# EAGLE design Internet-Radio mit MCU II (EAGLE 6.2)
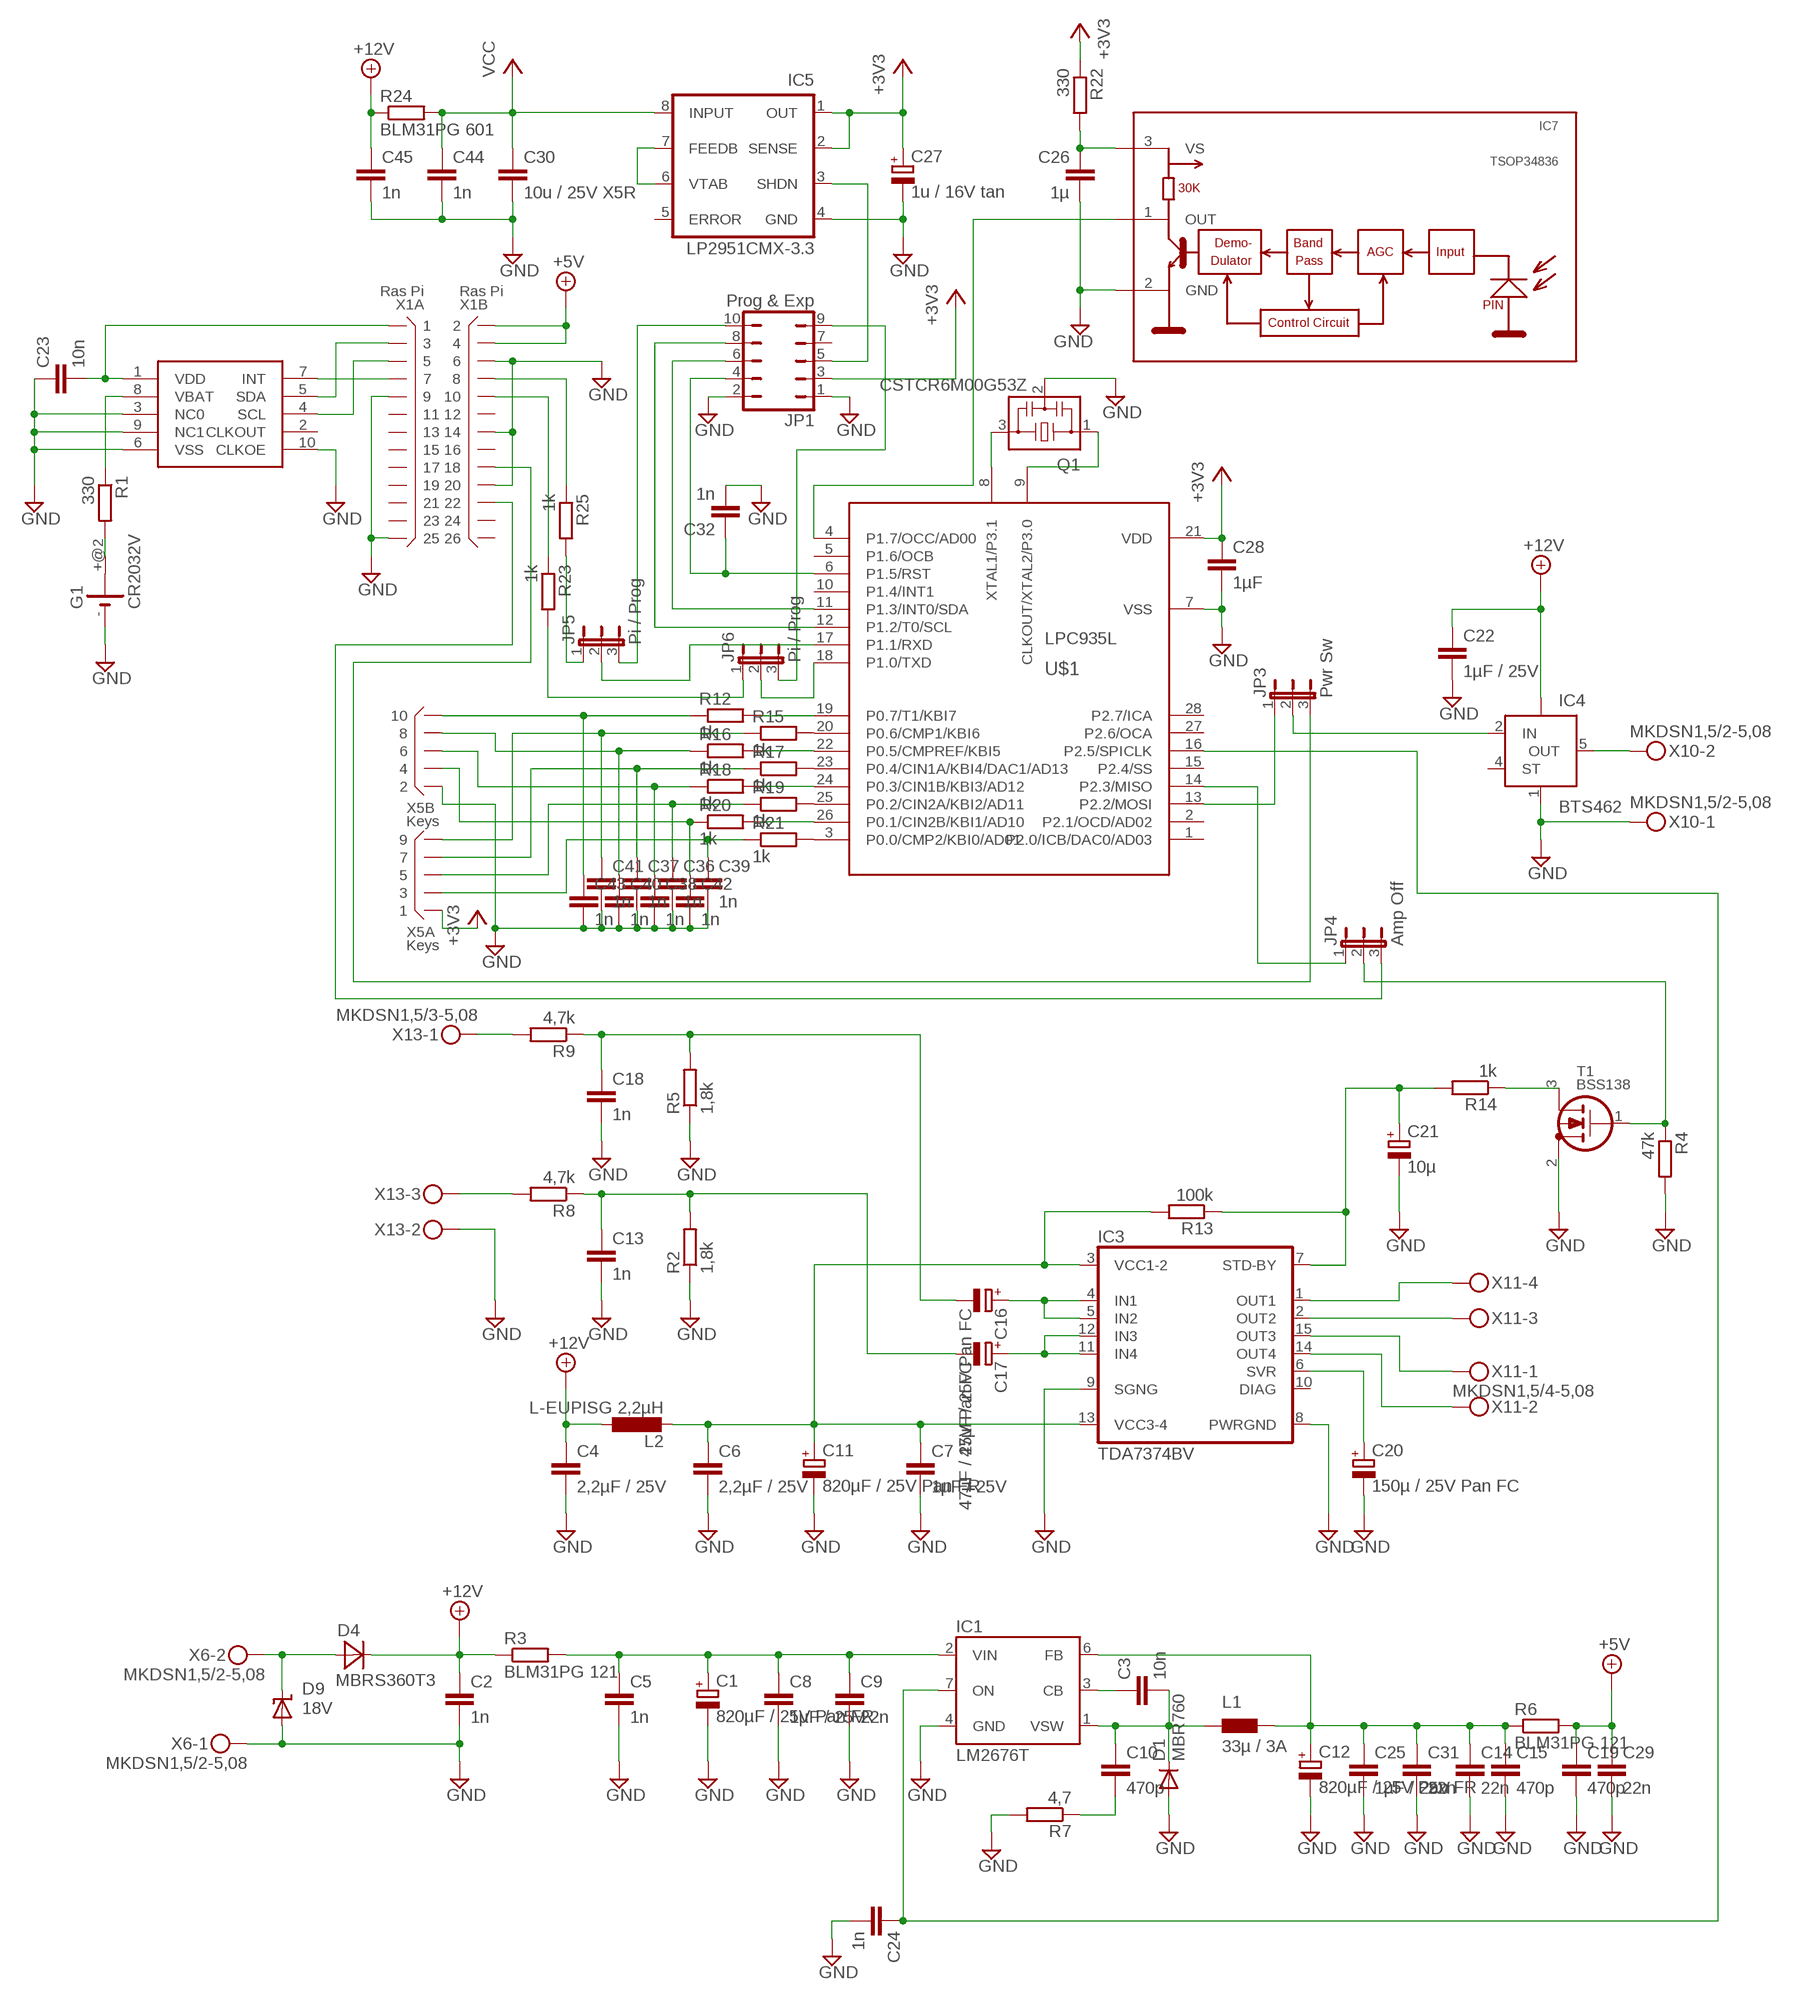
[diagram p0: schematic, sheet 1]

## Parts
C1  820µF / 25V Pan FR  CPOL-EUTT5D10  [TT5D10]
C2  1n  C-EUC0805  [C0805]
C3  10n  C-EUC0805  [C0805]
C4  2,2µF / 25V  C-EUC0805  [C0805]
C5  1n  C-EUC0805  [C0805]
C6  2,2µF / 25V  C-EUC0805  [C0805]
C7  1µF / 25V  C-EUC0805  [C0805]
C8  1µF / 25V  C-EUC0805  [C0805]
C9  22n  C-EUC0805  [C0805]
C10  470p  C-EUC0805  [C0805]
C11  820µF / 25V Pan FR  CPOL-EUTT5D10  [TT5D10]
C12  820µF / 25V Pan FR  CPOL-EUTT5D10  [TT5D10]
C13  1n  C-EUC0805  [C0805]
C14  22n  C-EUC0805  [C0805]
C15  470p  C-EUC0805  [C0805]
C16  47µF / 25V Pan FC  CPOL-EUE2.5-5  [E2,5-5]
C17  47µF / 25V Pan FC  CPOL-EUE2.5-5  [E2,5-5]
C18  1n  C-EUC0805  [C0805]
C19  470p  C-EUC0805  [C0805]
C20  150µ / 25V Pan FC  CPOL-EUE3.5-8  [E3,5-8]
C21  10µ  CPOL-EUE2.5-5  [E2,5-5]
C22  1µF / 25V  C-EUC0805  [C0805]
C23  10n  C-EUC0805  [C0805]
C24  1n  C-EUC0805  [C0805]
C25  1µF / 25V  C-EUC0805  [C0805]
C26  1µ  C-EUC0805  [C0805]
C27  1u / 16V tan  CPOL-EUCT3216  [CT3216]
C28  1µF  C-EUC0805  [C0805]
C29  22n  C-EUC0805  [C0805]
C30  10u / 25V X5R  C-EUC1206  [C1206]
C31  22n  C-EUC0805  [C0805]
C32  1n  C-EUC0805  [C0805]
C36  1n  C-EUC0603  [C0603]
C37  1n  C-EUC0603  [C0603]
C38  1n  C-EUC0603  [C0603]
C39  1n  C-EUC0603  [C0603]
C40  1n  C-EUC0603  [C0603]
C41  1n  C-EUC0603  [C0603]
C42  1n  C-EUC0603  [C0603]
C43  1n  C-EUC0603  [C0603]
C44  1n  C-EUC0805  [C0805]
C45  1n  C-EUC0805  [C0805]
D1  MBR760  DIODE-TO220V  [TO220ACS]
D4  MBRS360T3  [SMC]
D9  18V  SUPPRESSOR-SMBJ  [SMBJ]
G1  CR2032V  [CR2032V]
IC1  LM2676T  [TO220-7]
IC3  TDA7374BV  [MULTIWATT-15V]
IC4  BTS462  BTS428L2  [TO252-5-11]
IC5  LP2951CMX-3.3  [SO-08]
IC7  TSOP34836  [TSOP348]
JP1  Prog & Exp  JP5Q  [JP5Q]
JP3  Pwr Sw  JP2E  [JP2]
JP4  Amp Off  JP2E  [JP2]
JP5  Pi / Prog  JP2E  [JP2]
JP6  Pi / Prog  JP2E  [JP2]
L1  33µ / 3A  PIS4728  [PIS4728]
L2  L-EUPISG 2,2µH  L-EUPISG  [PISG]
Q1  CSTCR6M00G53Z  [CSTCR6M]
R1  330  R-EU_R1206  [R1206]
R2  1,8k  R-EU_R1206  [R1206]
R3  BLM31PG 121  R-EU_R1206  [R1206]
R4  47k  R-EU_R1206  [R1206]
R5  1,8k  R-EU_R1206  [R1206]
R6  BLM31PG 121  R-EU_R1206  [R1206]
R7  4,7  R-EU_R1206  [R1206]
R8  4,7k  R-EU_R1206  [R1206]
R9  4,7k  R-EU_R1206  [R1206]
R12  1k  R-EU_R1206  [R1206]
R13  100k  R-EU_R1206  [R1206]
R14  1k  R-EU_R1206  [R1206]
R15  1k  R-EU_R1206  [R1206]
R16  1k  R-EU_R1206  [R1206]
R17  1k  R-EU_R1206  [R1206]
R18  1k  R-EU_R1206  [R1206]
R19  1k  R-EU_R1206  [R1206]
R20  1k  R-EU_R1206  [R1206]
R21  1k  R-EU_R1206  [R1206]
R22  330  R-EU_R1206  [R1206]
R23  1k  R-EU_R1206  [R1206]
R24  BLM31PG 601  R-EU_R1206  [R1206]
R25  1k  R-EU_R1206  [R1206]
T1  BSS138  [SOT23]
U$1  LPC935L  [PLCC28]
U$4  RV3029-C2  [MC_RTC]
X1  Ras Pi  X13X2  [X26N-IDC]
X5  Keys  X05X2  [X10N-IDC]
X6  MKDSN1,5/2-5,08  [MKDSN1,5/2-5,08]
X10  MKDSN1,5/2-5,08  [MKDSN1,5/2-5,08]
X11  MKDSN1,5/4-5,08  [MKDSN1,5/4-5,08]
X13  MKDSN1,5/3-5,08  [MKDSN1,5/3-5,08]

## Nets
+3V3: C27.+ C28.1 IC5.1(OUT) IC5.2(SENSE) JP1.3 R22.1 U$1.21(VDD) X5.1
+5V: C19.1 C29.1 R6.2 X1.2 X1.4
+12V: C2.1 C4.1 C22.1 C45.1 D4.C IC4.TAB(VBB) L2.1 R3.1 R24.1
GND: C1.- C2.2 C4.2 C5.2 C6.2 C7.2 C8.2 C9.2 C11.- C12.- C13.2 C14.2 C15.2 C18.2 C19.2 C20.- C21.- C22.2 C23.1 C24.2 C25.2 C26.2 C27.- C28.2 C29.2 C30.2 C31.2 C32.2 C36.2 C37.2 C38.2 C39.2 C40.2 C41.2 C42.2 C43.2 C44.2 C45.2 D1.A D9.A G1.- IC1.4(GND) IC3.8(PWRGND) IC3.9(SGNG) IC4.1(GND) IC5.4(GND) IC7.2(GND) JP1.1 JP1.2 Q1.2 R2.1 R4.2 R5.1 R7.2 T1.2(S) U$1.7(VSS) U$4.3(NC0) U$4.6(VSS) U$4.9(NC1) U$4.10(CLKOE) X1.6 X1.9 X1.14 X1.20 X1.25 X5.2 X6.1 X10.1 X13.2
N$1: C1.+ C5.1 C8.1 C9.1 IC1.2(VIN) R3.2
N$2: C3.2 C10.1 D1.C IC1.1(VSW) L1.P$1
N$3: IC3.1(OUT1) X11.4
N$4: C3.1 IC1.3(CB)
N$5: IC3.2(OUT2) X11.3
N$6: IC3.15(OUT3) X11.1
N$7: IC3.14(OUT4) X11.2
N$8: C6.1 C7.1 C11.+ IC3.3(VCC1-2) IC3.13(VCC3-4) L2.2 R13.2
N$9: D4.A D9.C X6.2
N$10: C20.+ IC3.6(SVR)
N$11: G1.+@2(+) R1.2
N$12: C16.- C18.1 R5.2 R9.1
N$13: R9.2 X13.1
N$14: C13.1 C17.- R2.2 R8.1
N$15: C10.2 R7.1
N$16: R8.2 X13.3
N$17: C12.+ C14.1 C15.1 C25.1 C31.1 IC1.6(FB) L1.P$2 R6.1
N$18: C21.+ IC3.7(STD-BY) R13.1 R14.2
N$20: IC4.5(OUT) X10.2
N$23: R14.1 T1.3(D)
N$24: C16.+ IC3.4(IN1) IC3.5(IN2)
N$25: JP4.2 R4.1 T1.1(G)
N$26: C17.+ IC3.11(IN4) IC3.12(IN3)
N$27: JP3.1 U$1.13(P2.2/MOSI)
N$28: C24.1 IC1.7(ON) U$1.16(P2.5/SPICLK)
N$29: R1.1 U$4.8(VBAT)
N$30: Q1.3 U$1.8(XTAL1/P3.1)
N$31: Q1.1 U$1.9(CLKOUT/XTAL2/P3.0)
N$32: R12.2 U$1.19(P0.7/T1/KBI7)
N$33: R15.2 U$1.20(P0.6/CMP1/KBI6)
N$34: R16.2 U$1.22(P0.5/CMPREF/KBI5)
N$35: R18.2 U$1.24(P0.3/CIN1B/KBI3/AD12)
N$36: R20.2 U$1.26(P0.1/CIN2B/KBI1/AD10)
N$37: R21.2 U$1.3(P0.0/CMP2/KBI0/AD01)
N$38: R19.2 U$1.25(P0.2/CIN2A/KBI2/AD11)
N$39: R17.2 U$1.23(P0.4/CIN1A/KBI4/DAC1/AD13)
N$40: C26.1 IC7.3(VS) R22.2
N$41: IC5.6(VTAB) IC5.7(FEEDB)
N$42: C38.1 R18.1 X5.6
N$43: C36.1 R19.1 X5.5
N$44: C42.1 R20.1 X5.4
N$45: C39.1 R21.1 X5.3
N$46: C43.1 R12.1 X5.10
N$47: C41.1 R15.1 X5.9
N$48: C40.1 R16.1 X5.8
N$49: C37.1 R17.1 X5.7
N$50: C23.2 U$4.1(VDD) X1.1
N$51: JP5.1 R25.2
N$52: IC7.1(OUT) U$1.4(P1.7/OCC/AD00)
N$53: JP6.1 R23.2
N$54: R23.1 X1.10
N$55: R25.1 X1.8
N$56: C32.1 JP1.4 U$1.6(P1.5/RST)
N$57: IC5.3(SHDN) JP1.5
N$58: IC4.2(IN) JP3.2
N$59: JP3.3 X1.18
N$60: JP4.3 X1.22
N$61: JP6.2 U$1.18(P1.0/TXD)
N$62: JP4.1 U$1.14(P2.3/MISO)
N$63: JP5.2 U$1.17(P1.1/RXD)
P1.0: JP1.9 JP6.3
P1.1: JP1.10 JP5.3
P1.2: JP1.8 U$1.12(P1.2/T0/SCL)
P1.3: JP1.6 U$1.11(P1.3/INT0/SDA)
P1.4: U$4.5(SDA) X1.3
P1.5: U$4.4(SCL) X1.5
P1.6: U$4.7(INT) X1.7
VCC: C30.1 C44.1 IC5.8(INPUT) R24.2
Unconnected: G1.+ IC3.10(DIAG) IC4.4(ST) IC5.5(ERROR) JP1.7 U$1.1(P2.0/ICB/DAC0/AD03) U$1.2(P2.1/OCD/AD02) U$1.5(P1.6/OCB) U$1.10(P1.4/INT1) U$1.15(P2.4/SS) U$1.27(P2.6/OCA) U$1.28(P2.7/ICA) U$4.2(CLKOUT) X1.11 X1.12 X1.13 X1.15 X1.16 X1.17 X1.19 X1.21 X1.23 X1.24 X1.26

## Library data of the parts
C1 C11 C12 C16 C17 C20 C21 C27 = rcl:CPOL-EU: POLARIZED CAPACITOR, European symbol
C2-C10 C13-C15 C18 C19 C22-C26 C28-C32 C36-C45 = rcl:C-EU: CAPACITOR, European symbol
D1 = diode:DIODE-: DIODE
D4 = diode:MBRS360T3: Surface Mount Schottky Power Rectifier
D9 = diode:SUPPRESSOR-: Suppressor diode
G1 = battery:CR2032V: LI BATTERY Varta
IC1 = v-reg-3:LM2676: National Semiconductor 3.0A "Simple Switcher"(c) 260kHz, Vout 1.2-37V, Vin 40V, 150mOhm DMOS switch, 50µA standby current
IC3 = st-tda737X:TDA7374B
IC4 = infineon:BTS428L2: Smart High-Side Power Switch One Channel: 60mOhm Status Feedback Source: Source: www.infineon.com .. BTS428L2_20030912.pdf; OC_FARNELL: unknown; OC_NEWARK: unknown
IC5 = v-reg:LP2951?*: Series of Adjustable Micropower Voltage Regulators Source: http://cache.national.com/ds/LP/LP2950.pdf
IC7 = vishay-1:TSOP348*: IR Receiver Modules for Remote Control Systems http://www.vishay.com/ir-receiver-modules/
JP1 = jumper:JP5Q: JUMPER
JP3-JP6 = jumper:JP2E: JUMPER
L1 = inductor-fastron:PIS4728: Fastron SMD Power Inductors
L2 = Inductor-Fastron (2):L-EU
Q1 = murata-filter:CSTCR: Resonator Source: murata.co.jp; MPN: CSTCR6M00G53-R0; OC_FARNELL: 1170434; OC_NEWARK: 25M8759
R1 R2 R4 R5 R7-R9 R13 R14 R22 R23 R25 = rcl:R-EU_: RESISTOR, European symbol
R3 R6 R12 R15-R21 R24 = resistor:R-EU_: RESISTOR, European symbol
T1 = transistors:BSS138: BSS138: N-channel enhancement MOSFET (ON Semiconductor) 50V Uds, 200mA Id, 225mW Ptot, 3.5&Omega; Rdson
U$1 = nxp:LPC935
U$4 = MicroCrystal:RV3029-C2
X1 = connectors:X13X2: Connector 2x13 pins
X5 = connectors:X05X2: Connector 2x5 pins
X6 X10 = con-phoenix-508:MKDSN1,5/2-5,08: MKDSN 1,5/ 2-5,08 Printklemme; MPN: MKDSN 1,5/2-5.08; OC_FARNELL: 1792903; OC_NEWARK: 30M2397
X11 = con-phoenix-508:MKDSN1,5/4-5,08: MKDSN 1,5/ 4-5,08 Printklemme Nennstrom: 13,5 A Nennspannung: 250 V Rastermaß: 5,08 mm Polzahl: 4 Anschlussart: Schraubanschluss Montage: Löten Anschlussrichtung Leiter/Platine: 0 ° Artikelnummer: 1729144 Source: http://eshop.phoenixcontact.com .. 1729144.pdf
X13 = con-phoenix-508:MKDSN1,5/3-5,08: MKDSN 1,5/ 3-5,08 Printklemme Nennstrom: 13,5 A Nennspannung: 250 V Rastermaß: 5,08 mm Polzahl: 3 Anschlussart: Schraubanschluss Montage: Löten Anschlussrichtung Leiter/Platine: 0 ° Artikelnummer: 1729131 Source: http://eshop.phoenixcontact.com .. 1729131.pdf; MPN: SMKDSN1,5/3-5,08; OC_FARNELL: 1792904; OC_NEWARK: 70R0299

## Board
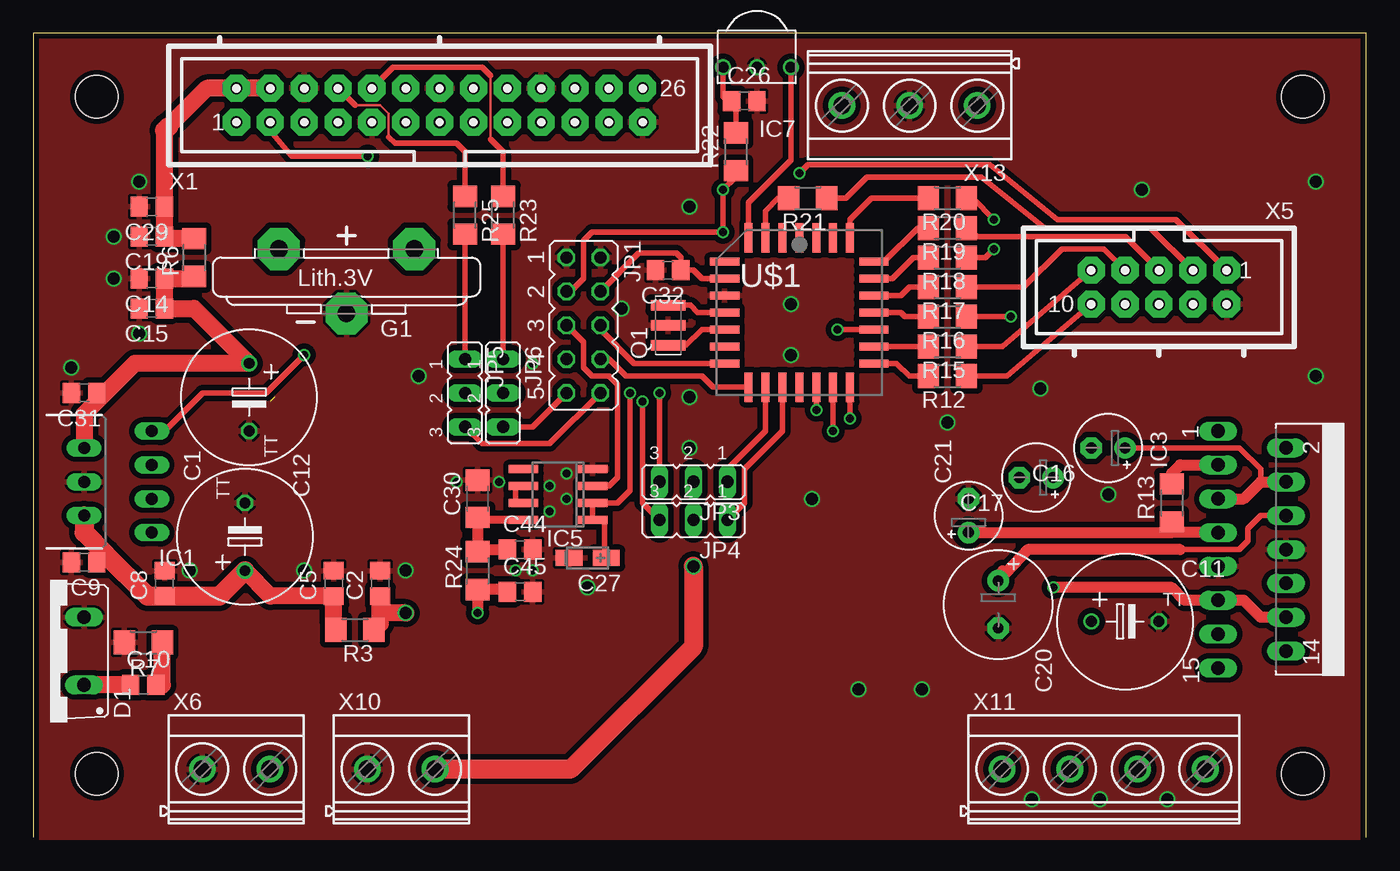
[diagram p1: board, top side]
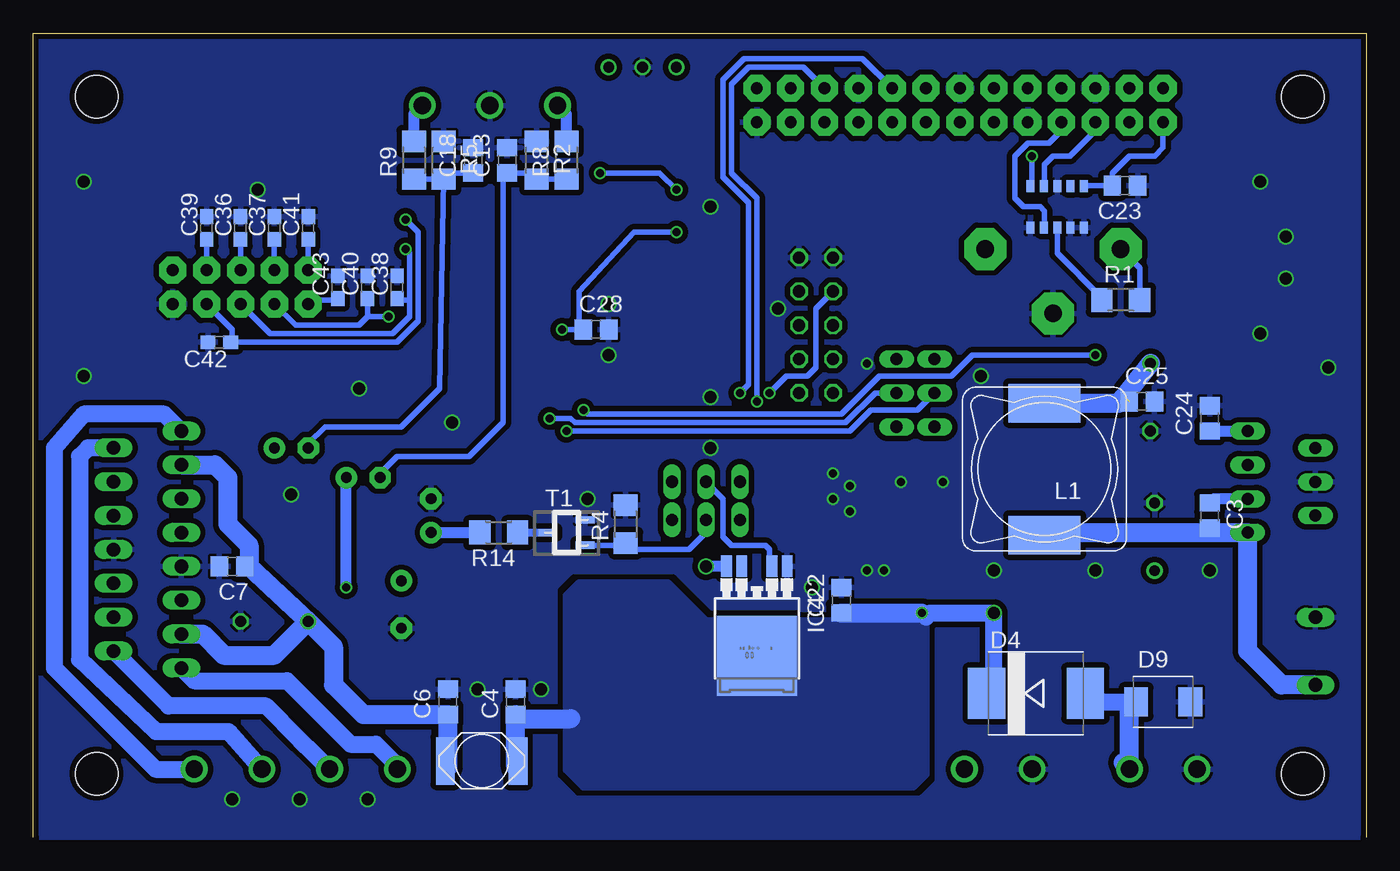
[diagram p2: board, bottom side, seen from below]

Size 100 x 60.33 mm. Coordinates in mm from the lower left corner, seen from the top.
Outline: 100,0 100,60.33 0,60.33 0,0
Copper layers (1*16): Top 0.035mm / dielectric 1.5mm / Bottom 0.035mm
Design rules: minimum track width 0.15mm, minimum drill 0.3mm, track to track 0.15mm, track to pad 0.15mm, pad to pad 0.15mm, via to via 0.15mm, smd to smd 0.15mm, copper to edge 0.3mm, drill to drill 0.2mm, minimum pad ring 0.2mm, minimum via ring 0.15mm, stop-mask expansion 0.075mm, vias tented up to drill 0mil, thermal gap 0.2mm
Holes 3.2 mm at 4.76,4.76 4.76,55.56 95.25,55.56 95.25,4.76

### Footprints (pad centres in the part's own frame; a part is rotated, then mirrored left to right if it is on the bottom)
TT5D10 = drill 0.813: + -2.54,0 | drill 0.813 octagon: - 2.54,0
C0805 = smd 1.3 x 1.5: 1 -0.95,0; 2 0.95,0
E2,5-5 = drill 0.813 pad 1.6: + -1.27,0 | drill 0.813 pad 1.6 octagon: - 1.27,0
E3,5-8 = drill 0.813 pad 1.6: + -1.778,0 | drill 0.813 pad 1.6 octagon: - 1.778,0
CT3216 = smd 2 x 1.2: + -1.4,0; - 1.4,0
C1206 = smd 1.6 x 1.8: 1 -1.4,0; 2 1.4,0
C0603 = smd 1.1 x 1: 1 -0.85,0; 2 0.85,0
TO220ACS = drill 1.016 long: A 2.54,-2.54; C -2.54,-2.54
SMC = smd 2.8 x 3.8: A 3.7,0; C -3.7,0
SMBJ = smd 1.78 x 2.16: A 2.04,0; C -2.03,0
CR2032V = drill 1.321 pad 3.15 octagon: + -2.54,5.08; +@2 -2.54,-5.08; - 2.286,0
TO220-7 = drill 0.9 long: 1 -3.81,-5.08; 2 -2.54,0; 3 -1.27,-5.08; 4 0,0; 5 1.27,-5.08; 6 2.54,0; 7 3.81,-5.08
MULTIWATT-15V = drill 1.016 long: 1 -8.89,-7.62; 2 -7.62,-2.54; 3 -6.35,-7.62; 4 -5.08,-2.54; 5 -3.81,-7.62; 6 -2.54,-2.54; 7 -1.27,-7.62; 8 0,-2.54; 9 1.27,-7.62; 10 2.54,-2.54; 11 3.81,-7.62; 12 5.08,-2.54; 13 6.35,-7.62; 14 7.62,-2.54; 15 8.89,-7.62
TO252-5-11 = smd 0.8 x 1.6: 1 -2.28,-5.41; 2 -1.14,-5.41; 4 1.14,-5.41; 5 2.28,-5.41 | smd 6 x 6: TAB 0,1.3
SO-08 = smd 0.6 x 2.2: 1 -1.905,-2.6; 2 -0.635,-2.6; 3 0.635,-2.6; 4 1.905,-2.6; 5 1.905,2.6; 6 0.635,2.6; 7 -0.635,2.6; 8 -1.905,2.6
TSOP348 = drill 0.8: 1 -2.54,0; 2 0,0; 3 2.54,0
JP5Q = drill 0.914 octagon: 1 -5.08,-1.27; 2 -5.08,1.27; 3 -2.54,-1.27; 4 -2.54,1.27; 5 0,-1.27; 6 0,1.27; 7 2.54,-1.27; 8 2.54,1.27; 9 5.08,-1.27; 10 5.08,1.27
JP2 = drill 0.914 long: 1 -2.54,0; 2 0,0; 3 2.54,0
PIS4728 = smd 5.4 x 2.9: P$1 0,4.95; P$2 0,-4.95
PISG = smd 1.4 x 3.56: 1 -2.73,0; 2 2.73,0
CSTCR6M = smd 0.8 x 2.6: 1 -1.5,0; 2 0,0; 3 1.5,0
R1206 = smd 1.6 x 1.803: 1 -1.422,0; 2 1.422,0
SOT23 = smd 0.55 x 1.4: 1 0.95,1.4; 2 -0.95,1.4; 3 0,-1.4
PLCC28 = smd 0.6 x 2.2: 1 0,5.6; 2 -1.27,5.6; 3 -2.54,5.6; 4 -3.81,5.6; 12 -3.81,-5.6; 13 -2.54,-5.6; 14 -1.27,-5.6; 15 0,-5.6; 16 1.27,-5.6; 17 2.54,-5.6; 18 3.81,-5.6; 26 3.81,5.6; 27 2.54,5.6; 28 1.27,5.6 | smd 2.2 x 0.6: 5 -5.6,3.81; 6 -5.6,2.54; 7 -5.6,1.27; 8 -5.6,0; 9 -5.6,-1.27; 10 -5.6,-2.54; 11 -5.6,-3.81; 19 5.6,-3.81; 20 5.6,-2.54; 21 5.6,-1.27; 22 5.6,0; 23 5.6,1.27; 24 5.6,2.54; 25 5.6,3.81
MC_RTC = smd 0.6 x 0.899: 1 -2,-1.549; 2 -1,-1.549; 3 0,-1.549; 4 1,-1.549; 5 2,-1.549; 6 2,1.549; 7 1,1.549; 8 0,1.549; 9 -1,1.549; 10 -2,1.549
X26N-IDC = drill 0.889 pad 2.032 octagon: 1 -15.24,-1.27; 2 -15.24,1.27; 3 -12.7,-1.27; 4 -12.7,1.27; 5 -10.16,-1.27; 6 -10.16,1.27; 7 -7.62,-1.27; 8 -7.62,1.27; 9 -5.08,-1.27; 10 -5.08,1.27; 11 -2.54,-1.27; 12 -2.54,1.27; 13 0,-1.27; 14 0,1.27; 15 2.54,-1.27; 16 2.54,1.27; 17 5.08,-1.27; 18 5.08,1.27; 19 7.62,-1.27; 20 7.62,1.27; 21 10.16,-1.27; 22 10.16,1.27; 23 12.7,-1.27; 24 12.7,1.27; 25 15.24,-1.27; 26 15.24,1.27
X10N-IDC = drill 0.889 pad 2.032 octagon: 1 -5.08,-1.27; 2 -5.08,1.27; 3 -2.54,-1.27; 4 -2.54,1.27; 5 0,-1.27; 6 0,1.27; 7 2.54,-1.27; 8 2.54,1.27; 9 5.08,-1.27; 10 5.08,1.27
MKDSN1,5/2-5,08 = drill 1.3 pad 2: 1 -2.561,0.025; 2 2.519,0.025
MKDSN1,5/4-5,08 = drill 1.3 pad 2: 1 -7.641,0.025; 2 -2.561,0.025; 3 2.519,0.025; 4 7.599,0.025
MKDSN1,5/3-5,08 = drill 1.3 pad 2: 1 -7.641,0.025; 2 -2.561,0.025; 3 2.519,0.025

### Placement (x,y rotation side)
C1  15.88,22.54 90 top
C2  26.04,19.05 90 top
C3  11.75,24.13 270 bottom
C4  63.82,10.16 90 bottom
C5  22.54,19.05 90 top
C6  68.9,10.16 90 bottom
C7  85.09,20.32 180 bottom
C8  9.84,19.05 90 top
C9  3.81,20.64 180 top
C10  8.26,11.43 0 top
C11  81.92,16.19 0 top
C12  16.19,33.02 270 top
C13  64.45,50.8 90 bottom
C14  8.89,41.91 180 top
C15  8.89,39.69 180 top
C16  80.64,29.21 180 top
C17  75.25,26.99 180 top
C18  66.99,50.8 90 bottom
C19  8.89,45.09 180 top
C20  72.39,17.46 270 top
C21  70.17,24.13 90 top
C22  39.37,17.78 90 bottom
C23  18.1,48.9 180 bottom
C24  11.75,31.43 90 bottom
C25  16.83,32.7 0 bottom
C26  53.34,55.24 0 top
C27  41.59,20.95 180 top
C28  57.78,38.1 0 bottom
C29  8.89,47.31 180 top
C30  33.34,25.4 90 top
C31  3.81,33.34 180 top
C32  47.62,42.55 180 top
C36  84.45,45.72 90 bottom
C37  81.92,45.72 90 bottom
C38  72.71,41.27 90 bottom
C39  87,45.72 90 bottom
C40  74.93,41.27 90 bottom
C41  79.38,45.72 90 bottom
C42  86.04,37.15 180 bottom
C43  77.15,41.27 90 bottom
C44  36.51,21.59 0 top
C45  36.51,18.41 0 top
D1  1.27,13.97 90 top
D4  24.77,10.79 0 bottom
D9  15.24,10.16 0 bottom
G1  23.5,41.59 270 top
IC1  3.81,26.67 90 top
IC3  96.52,21.59 270 top
IC4  45.72,14.92 180 bottom
IC5  39.37,25.72 90 top
IC7  54.29,57.78 180 top
JP1  41.27,38.42 270 top
JP3  49.53,26.67 180 top
JP4  49.53,23.81 180 top
JP5  32.38,33.34 270 top
JP6  35.24,33.34 270 top
L1  24.13,27.62 180 bottom
L2  66.36,5.71 180 bottom
Q1  47.62,38.42 90 top
R1  18.41,40.32 0 bottom
R2  62.23,50.8 270 bottom
R3  24.13,15.56 180 top
R4  55.56,23.5 90 bottom
R5  69.22,50.8 270 bottom
R6  12.06,43.5 90 top
R7  8.26,14.61 180 top
R8  60.01,50.8 90 bottom
R9  71.44,50.8 90 bottom
R12  68.58,34.61 180 top
R13  85.41,25.08 90 top
R14  65.09,22.86 180 bottom
R15  68.58,36.83 180 top
R16  68.58,39.05 180 top
R17  68.58,41.27 180 top
R18  68.58,43.5 180 top
R19  68.58,45.72 180 top
R20  68.58,47.94 180 top
R21  58.1,47.94 180 top
R22  52.7,51.44 90 top
R23  35.24,46.67 270 top
R24  33.34,20 90 top
R25  32.38,46.67 270 top
T1  60.01,22.86 270 bottom
U$1  57.47,39.37 0 top
U$4  23.18,47.31 180 bottom
X1  30.48,54.93 0 top
X5  84.45,41.27 180 top
X6  15.24,5.08 0 top
X10  27.62,5.08 0 top
X11  80.33,5.08 0 top
X13  63.18,54.93 180 top

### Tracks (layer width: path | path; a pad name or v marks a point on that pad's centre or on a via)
+3V3  (via drill 0.6)
  Top 0.406: JP1.3 40.32,40.96 41.27,41.91 41.27,44.77 41.91,45.4 v51.75,45.4 v51.75,48.58 52.7,49.53 R22.1 | 43.18,20.95 C27.+ 42.86,21.59 42.86,23.81 IC5.1 IC5.2 43.81,25.08 44.77,26.04 v44.77,33.34 | X5.1 85.72,46.35 76.83,46.35 71.75,50.48 58.1,50.48 v57.47,49.85 | U$1.21 v60.33,38.1
  Bottom 0.406: v57.47,49.85 53.02,49.85 v51.75,48.58 | v60.33,38.1 59.05,38.1 | 59.05,38.1 59.05,40.96 54.93,45.4 v51.75,45.4 | v44.77,33.34 43.5,34.61 41.91,34.61 41.27,35.24 41.27,39.69 JP1.3 | C28.1 59.05,38.1
+5V
  Top 1.27: X1.4 X1.2 13.02,56.2 10.16,53.34 9.84,53.02 C29.1 C19.1 10.01,44.92 R6.2
  Top 1.422: 10.16,53.34 9.84,53.02
+12V  (via drill 0.6, 0.9)
  Top 0.813: v33.34,16.83 R24.1 35.4,18.58 C45.1
  Top 1.27: R3.1 26.04,16.04 26.04,16.83 | 26.04,16.83 C2.1 | v27.94,16.83 26.04,16.83
  Bottom 0.813: v33.34,16.83 33.02,16.51 | L2.1 63.82,5.27 | C4.1 63.5,8.89
  Bottom 1.27: 33.02,16.51 32.7,16.83 v27.94,16.83 27.94,11.32 D4.C
  Bottom 1.422: C22.1 v33.34,16.83 | 63.82,5.27 C4.1 | 63.5,8.89 59.69,8.89
  pour Bottom (no thermals): 38.42,16.83 39.05,16.19 49.53,16.19 52.39,19.05 59.05,19.05 60.01,18.1 60.01,5.08 58.74,3.81 33.97,3.81 33.02,4.76 33.02,16.83
GND  (via drill 0.6, 0.9)
  other vias: 61.91,11.11 66.67,11.11 20.32,20 27.94,20 80.01,2.86 85.09,2.86 74.93,2.86 56.83,36.2 56.83,40.01 49.21,47.31 96.2,34.61 96.2,49.21 58.42,25.4 75.56,33.66 49.21,33.02 40.01,27.3 38.73,26.35 38.73,24.45 40.01,25.4 36.2,20 37.47,20 28.89,34.61 49.21,29.21 41.59,18.73 31.75,26.67 68.58,31.11 37.47,35.56 34.92,26.67 44.13,39.69 83.19,48.58 80.64,25.72 7.94,37.78 6.03,41.91 6.03,45.09 7.94,49.21 2.86,35.24 11.75,20
  pour Bottom (isolate 0.406, rank 2): 0,0 100.33,0 100.01,60.33 0,60.33
  pour Top (isolate 0.406): 0,60.33 100.01,60.33 100.33,0 0,0
N$1
  Top 1.27: R3.2 22.54,16.03 C5.1 17.78,18.1 C1.+ | C9.1 5.4,21.27
  Top 1.422: IC1.2 3.81,22.86 5.4,21.27 8.57,18.1 C8.1 11.43,18.1 13.97,18.1 C1.+
N$2
  Top 1.27: C10.1 D1.C
  Bottom 0.813: C3.2 11.43,22.86 IC1.1
  Bottom 1.422: D1.C 6.35,11.43 8.89,13.97 IC1.1 24,22.86 L1.P$1
N$3
  Bottom 1.27: IC3.1 90.17,31.75 96.2,31.75 98.42,29.21 98.42,12.7 90.83,5.11 X11.4
N$4
  Bottom 0.406: 11.43,25.4
  Bottom 0.813: IC1.3 11.43,25.4 | C3.1 11.43,25.4
N$5
  Bottom 1.27: X11.3 85.36,7.94 90.81,7.94 96.52,13.34 96.52,28.57 95.89,29.21 IC3.2
N$6
  Bottom 1.27: IC3.15 87.95,11.75 80.96,11.75 76.2,6.99 74.3,6.99 72.71,5.4 72.71,5.08 | X11.1 72.71,5.08 | 72.71,5.08
N$7
  Bottom 1.27: X11.2 77.79,5.13 80.01,7.3 82.55,9.84 89.85,9.84 IC3.14
N$8
  Top 0.813: R13.2 85.41,27.3 86.04,27.94 IC3.3
  Bottom 0.813: L2.2 68.9,5.27 | C7.1 83.82,20.32
  Bottom 1.422: 68.9,5.27 C6.1 75.25,9.21 77.47,11.43 77.47,14.29 C11.+ | IC3.3 86.36,27.94 85.41,26.99 85.41,23.5 83.82,21.91 83.82,20.32 C11.+ | IC3.13 87.31,15.24 85.72,13.65 81.92,13.65 C11.+
N$9
  Bottom 1.27: D4.A 20.43,10.16 D9.C
  Bottom 1.422: X6.2 17.78,5.13 | 17.78,5.13 17.78,9.84 17.46,10.16 D9.C 17.14,10.16 | 17.78,5.13 18.24,5.59
N$10
  Top 0.406: IC3.6 92.08,24.13 91.12,23.18 91.12,22.23 90.49,21.59 86.04,21.59
  Top 0.813: 86.04,21.59 74.61,21.59 C20.+ 72.71,20
N$11
  Bottom 0.406: R1.2 16.99,42.71 G1.+@2
N$12
  Bottom 0.406: R5.2 69.53,33.66 72.39,30.8 78.11,30.8 79.38,29.53 C16.- | R5.2 68.75,49.85 C18.1 | R5.2 R9.1
N$13
  Bottom 0.813: R9.2 71.44,54.29 X13.1
N$14
  Bottom 0.406: R8.1 R2.2 62.7,49.85 C13.1 64.77,49.53 64.77,31.11 67.31,28.57 72.71,28.57 73.98,27.3 C17.-
N$15
  Top 1.27: C10.2 9.68,11.43 R7.1
N$16
  Bottom 0.813: R8.2 60.01,54.29 60.62,54.9 X13.3
N$17  (1 unrouted)
  Top 1.27: 4.76,32.7 7.62,35.56 C12.+ 12.06,39.69 C15.1 C14.1 11.9,41.91 R6.1 | IC1.6 3.81,31.75 4.76,32.7 | C31.1 4.76,32.7
  Bottom 0.813: 18.1,33.02 18.19,33.02
  Bottom 1.422: L1.P$2 18.55,32.57 18.19,33.02 C12.+
N$18
  Top 0.813: C21.+ 85.41,22.86 | 85.41,22.86 R13.1 | IC3.7 85.41,22.86
  Bottom 0.813: C21.+ R14.2
N$20  (via drill 0.9)
  Top 1.422: v49.53,20.32 49.53,14.29 40.3,5.1 X10.2
  Bottom 0.813: IC4.5 48.3,20.32 v49.53,20.32
N$23
  Bottom 0.61: R14.1 T1.3
N$24
  Top 0.406: C16.+ 90.49,29.21 92.08,27.62 92.08,26.67
  Top 0.813: IC3.5 90.81,25.4 92.08,26.67 IC3.4
N$25
  Bottom 0.406: JP4.2 49.53,22.86 50.8,21.59 55.08,21.59 R4.1 55.73,21.91 T1.1
N$26  (via drill 0.6)
  Top 0.813: IC3.12 92.08,16.51 90.81,17.78 IC3.11 86.36,17.78 85.41,18.73 v76.52,18.73
  Bottom 0.813: v76.52,18.73 C17.+
N$27
  Top 0.406: JP3.1 52.07,27.62 54.93,30.48 U$1.13 54.93,33.97
N$28  (via drill 0.6)
  Top 0.406: U$1.16 v58.74,32.07 | v20.32,36.2 17.46,33.34 12.7,33.34 9.84,30.48 IC1.7
  Bottom 0.406: v58.74,32.07 58.42,31.75 39.37,31.75 36.51,34.61 31.11,34.61 29.53,36.2 v20.32,36.2
  Bottom 0.813: C24.1 11.43,30.48 IC1.7
N$29
  Bottom 0.406: U$4.8 23.18,43.81 19.84,40.47 R1.1
N$30
  Top 0.406: U$1.8 49.85,39.37 49.3,39.92 Q1.3
N$31
  Top 0.406: U$1.9 50.16,38.1 48.98,36.92 Q1.1
N$32
  Top 0.406: U$1.19 64.77,35.56 65.72,34.61 R12.2
N$33
  Top 0.406: R15.2 U$1.20
N$34
  Top 0.406: U$1.22 65.09,39.37 65.41,39.05 R16.2
N$35
  Top 0.406: U$1.24 64.45,41.91 66.04,43.5 R18.2
N$36
  Top 0.406: U$1.26 61.28,46.35 62.87,47.94 R20.2
N$37
  Top 0.406: U$1.3 54.93,46.99 55.88,47.94 R21.2
N$38
  Top 0.406: U$1.25 63.82,43.18 66.36,45.72 R19.2
N$39
  Top 0.406: U$1.23 65.09,40.64 65.72,41.27 R17.2
N$40
  Top 0.406: R22.2 52.7,54.76 51.75,55.56 | IC7.3 51.75,55.56 | 51.75,55.56 C26.1
N$41
  Top 0.406: IC5.7 36.2,25.14 36.2,26.35 IC5.6
N$42  (via drill 0.6)
  Top 0.406: v72.07,44.13 71.44,43.5 R18.1
  Bottom 0.406: X5.6 82.23,37.78 73.03,37.78 71.75,39.05 71.75,40.32 | 71.75,40.32 71.75,43.81 v72.07,44.13 | C38.1 72.92,40.32 71.75,40.32
N$43
  Top 0.406: X5.5 81.92,45.09 70.8,45.09 70.17,45.72 R19.1
  Bottom 0.406: C36.1 X5.5
N$44  (via drill 0.6)
  Top 0.406: R20.1 70.48,47.94 v72.07,46.35
  Bottom 0.406: v72.07,46.35 71.12,45.4 71.12,38.73 72.71,37.15 85.09,37.15 | X5.4 85.09,38.1 85.09,37.15 | C42.1 85.09,37.15
N$45
  Top 0.406: R21.1 60.96,47.94 62.55,49.53 71.12,49.53 75.88,45.72 83.82,45.72 X5.3
  Bottom 0.406: C39.1 X5.3
N$46
  Top 0.406: X5.10 73.03,34.61 R12.1
  Bottom 0.406: X5.10 79.06,40.32 77.15,40.32 C43.1
N$47
  Top 0.406: X5.9 72.71,36.83 R15.1
  Bottom 0.406: X5.9 C41.1
N$48  (via drill 0.6)
  Top 0.406: v73.34,39.05 R16.1
  Bottom 0.406: X5.8 80.33,38.42 75.56,38.42 74.93,39.05 | 74.93,39.05 v73.34,39.05 | C40.1 74.93,39.05
N$49
  Top 0.406: R17.1 74.3,41.27 77.15,44.13 80.33,44.13 X5.7
  Bottom 0.406: C37.1 X5.7
N$50
  Bottom 0.406: U$4.1 21.14,48.9 | X1.1 15.24,51.75 15.88,51.12 17.78,51.12 19.05,49.85 C23.2 21.14,48.9 | 21.14,48.9 21.27,48.9
N$51
  Top 0.406: R25.2 JP5.1
N$52
  Top 0.406: U$1.4 53.66,47.62 56.83,50.8 IC7.1
N$53
  Top 0.406: JP6.1 R23.2
N$54
  Top 0.203: 34.29,57.15 34.29,52.39
  Top 0.406: X1.10 26.99,57.78 33.66,57.78 34.29,57.15 | R23.1 35.24,51.44 34.29,52.39
N$55
  Top 0.203: 26.67,52.54 26.67,54.29 26.04,54.93 24.13,54.93
  Top 0.406: X1.8 24.13,54.93 | R25.1 32.38,51.44 31.75,52.07 27.14,52.07 26.67,52.54
N$56
  Top 0.406: U$1.6 50.16,41.91 49.53,42.55 C32.1 | C32.1 | JP1.4 45.4,43.81 48.26,43.81 48.58,43.5 C32.1
N$57
  Top 0.406: JP1.5 41.27,37.15 41.27,35.24 41.91,34.61 43.18,34.61 43.81,33.97 43.81,26.99 43.18,26.35 IC5.3
N$58
  Bottom 0.406: JP3.2 48.26,25.4 48.26,22.54 47.62,21.91 45.09,21.91 44.77,21.59 44.77,20.52 IC4.2
N$59  (via drill 0.6)
  Top 0.406: v46.99,33.34 JP3.3
  Bottom 0.406: X1.18 37.78,58.42 46.67,58.42 48.26,56.83 48.26,49.53 46.35,47.62 46.35,33.97 v46.99,33.34
N$60  (via drill 0.6)
  Top 0.406: JP4.3 45.72,25.08 v45.72,32.7
  Bottom 0.406: X1.22 42.23,57.78 46.35,57.78 47.62,56.52 47.62,49.85 45.72,47.94 v45.72,32.7
N$61  (via drill 0.6)
  Top 0.406: v61.28,31.43 U$1.18
  Bottom 0.406: JP6.2 36.83,33.34 39.05,31.11 59.37,31.11 59.69,31.43 v61.28,31.43
N$62
  Top 0.406: JP4.1 53.34,25.08 53.34,27.62 56.2,30.48 U$1.14
N$63  (via drill 0.6)
  Top 0.406: v60.01,30.48 U$1.17
  Bottom 0.406: JP5.2 33.66,32.07 37.15,32.07 38.73,30.48 v60.01,30.48
P1.0
  Top 0.406: JP6.3 37.47,30.8 JP1.9
P1.1
  Top 0.406: JP5.3 33.66,29.53 38.73,29.53 JP1.10
P1.2
  Top 0.406: JP1.8 43.18,35.88 44.45,34.61 50.16,34.61 51,33.77 U$1.12
P1.3
  Top 0.406: JP1.6 42.55,38.1 45.09,35.56 U$1.11 52.07,35.56
P1.4  (via drill 0.6)
  Top 0.406: v25.08,51.12 19.37,51.12 17.78,53.02 X1.3
  Bottom 0.406: U$4.5 25.08,48.95 v25.08,51.12
P1.5
  Bottom 0.406: U$4.4 24.13,48.9 24.13,50.48 23.5,51.12 22.23,51.12 20.32,53.02 X1.5
P1.6
  Bottom 0.406: U$4.7 24.13,45.81 24.13,46.99 24.45,47.31 25.72,47.31 26.35,47.94 26.35,51.12 25.4,52.07 23.81,52.07 22.86,53.02 X1.7
VCC
  Top 0.61: IC5.8 33.66,23.81 33.47,24 C30.1
  Top 0.813: C30.1 R24.2 33.5,21.59 C44.1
